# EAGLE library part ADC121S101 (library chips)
Analogue to Digital Converter, 12 bit, 1 MSPS, Single, 2.7 V, 5.25 V, SOT-23
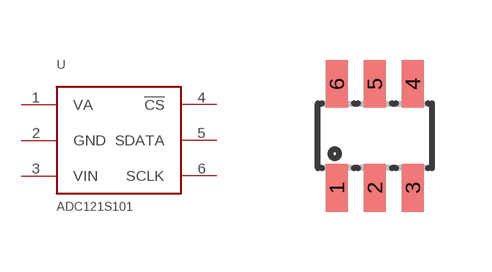
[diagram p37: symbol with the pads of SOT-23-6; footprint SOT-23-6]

Designator prefix -

## ADC121S101 (DIGIKEY: ADC121S101CIMF/NOPBCT-ND; MOUSER: 926-AD121S101CISDNPB; NEWARK: 96K6188)  [SOT-23-6]
1  VA
2  GND
3  VIN
4  !CS
5  SDATA
6  SCLK

## Footprint SOT-23-6 (pad centres in mm)
Small Outline Transistor
smd 0.55 x 1.2: 1 -0.95,-1.3; 2 0,-1.3; 3 0.95,-1.3; 4 0.95,1.3; 5 0,1.3; 6 -0.95,1.3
